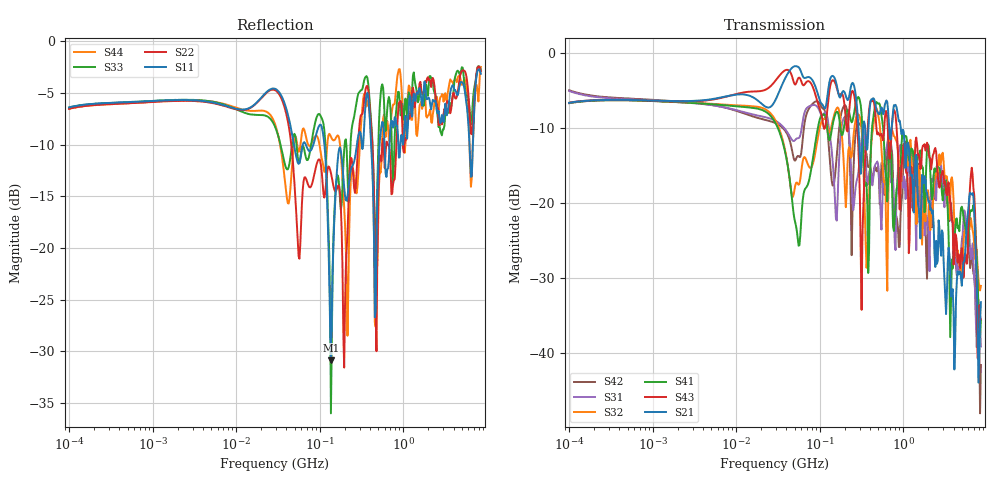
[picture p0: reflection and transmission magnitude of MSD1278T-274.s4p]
# MHz S MA R 50
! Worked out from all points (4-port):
!   498 points, 100 kHz to 8.5 GHz, reference 50 ohm
!   strongest paths, dB at 100 kHz, 1.698 MHz, 29.49 MHz, 500.7 MHz, 8.5 GHz:
!     S21: -6.6, -6.4, -6.3, -8.0, -33.2
!     S43: -6.6, -6.4, -3.7, -10.6, -35.5
!     S41: -6.7, -6.5, -9.3, -6.7, -35.7
!     S32: -6.7, -6.5, -8.9, -8.3, -31.0
!     S31: -5.1, -6.5, -9.0, -14.9, -39.1
!     S42: -5.0, -6.4, -9.3, -15.1, -41.5
!   lowest |S11| = -30.9 dB at 136.2 MHz (marker M1), VSWR 1.06, Z = 51.9 - j2.23 ohm
!   |S11| at or under -10 dB: 113.8 MHz to 278.8 MHz (165.1 MHz wide, 84.1 % of centre); 412.6 MHz to 520.6 MHz (108 MHz wide, 23.1 % of centre); 6.204 GHz to 6.825 GHz (620.2 MHz wide, 9.52 % of centre)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
0.1  0.4784 17.3  0.4659 17.6  0.5589 -15.6  0.4642 -163.4
     0.4659 17.6  0.471 17.4  0.4642 -163.4  0.5655 -15.4
     0.5589 -15.6  0.4642 -163.4  0.4775 17.4  0.4664 17.4
     0.4642 -163.4  0.5655 -15.4  0.4664 17.4  0.4704 17.6
98.93298  0.3909 -53.2  0.4949 -32.8  0.4152 8.2  0.3522 103.6
          0.4949 -32.8  0.2679 -26.4  0.3085 116.3  0.4657 -9.7
          0.4152 8.2  0.3085 116.3  0.4442 -31.0  0.4327 -42.7
          0.3522 103.6  0.4657 -9.7  0.4327 -42.7  0.3185 -31.2
136.2065  0.02859 -48.8  0.6914 -19.6  0.2512 -62.8  0.2853 49.6
          0.6914 -19.6  0.2304 -35.9  0.3148 40.1  0.158 -144.3
          0.2512 -62.8  0.3148 40.1  0.01586 -60.1  0.632 -20.2
          0.2853 49.6  0.158 -144.3  0.632 -20.2  0.3449 -28.7
317.0858  0.3272 -3.7  0.1918 -39.6  0.2692 -18.0  0.3933 -79.8
          0.1918 -39.6  0.4414 2.4  0.3109 -94.9  0.3301 -35.9
          0.2692 -18.0  0.3109 -94.9  0.5797 -14.8  0.01952 55.1
          0.3933 -79.8  0.3301 -35.9  0.01952 55.1  0.4263 8.9
417.0585  0.2895 -90.6  0.4927 -48.0  0.1466 -67.0  0.2835 18.0
          0.4927 -48.0  0.3626 -85.4  0.2621 30.1  0.151 -63.3
          0.1466 -67.0  0.2621 30.1  0.3842 -82.3  0.4845 -42.2
          0.2835 18.0  0.151 -63.3  0.4845 -42.2  0.3113 -92.2
2159.325  0.468 -173.2  0.09215 90.2  0.145 -174.4  0.1228 114.3
          0.09215 90.2  0.5999 -177.9  0.08801 172.0  0.0915 135.9
          0.145 -174.4  0.08801 172.0  0.6606 179.2  0.1682 124.8
          0.1228 114.3  0.0915 135.9  0.1682 124.8  0.4056 -175.1
8500  0.6952 -56.3  0.02193 -36.7  0.01113 -97.2  0.01646 -121.2
      0.02193 -36.7  0.7142 -57.7  0.02818 -136.2  0.008379 -56.8
      0.01113 -97.2  0.02818 -136.2  0.7266 -54.3  0.01684 -101.7
      0.01646 -121.2  0.008379 -56.8  0.01684 -101.7  0.7504 -47.5
